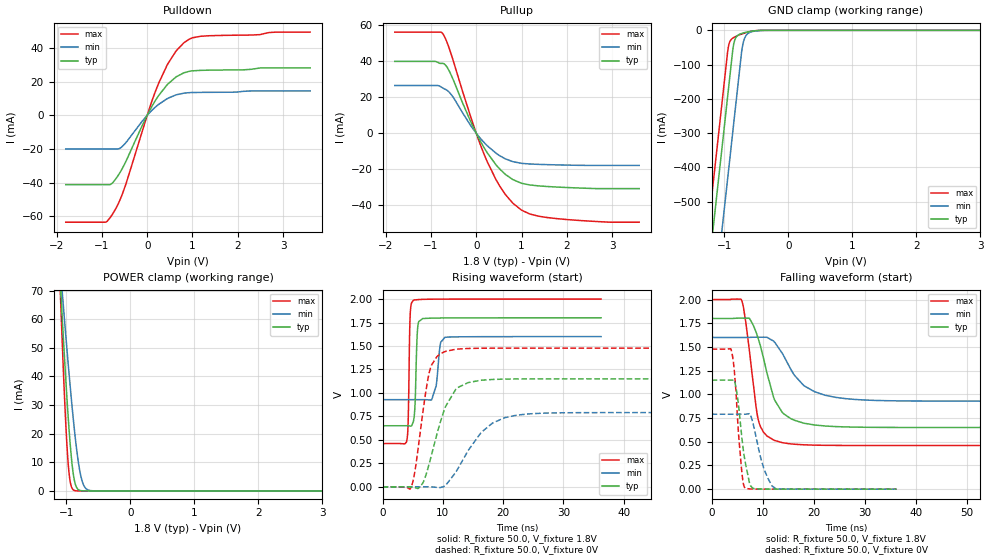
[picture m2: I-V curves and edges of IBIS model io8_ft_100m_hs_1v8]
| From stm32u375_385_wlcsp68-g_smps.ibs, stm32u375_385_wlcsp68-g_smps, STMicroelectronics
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[Model]   io8_ft_100m_hs_1v8
Model_type I/O
Polarity   Non-Inverting
Enable   Active-Low
| CAP_THRESHOLD on pad IOFT is "UDTCAPC" :
| Rising=30.0% of vddiom   Falling=70.0% of vddiom
| C_comp min and max val. don't necessarily correlate with the min and max pvt
| but are the smallest and greatest pad capacitance found.
| var   typ   min   max
C_comp   3.41155pF  3.41004pF  3.47580pF
|C_comp_pullup   1.91894pF  1.83594pF  2.09561pF
|C_comp_pulldown   1.49260pF  1.57410pF  1.38018pF
Vinl = 800.0mV
Vinh = 1.0V
Vmeas = 900.0mV   | Reference voltage for timing measurements
Cref  = 50.0pF   | Timing specification test load capacitance value
Rref  = 1.0MOhm   | Timing specification test load resistance value
Vref  = 990.0mV   | Timing specification test load voltage
[Model Spec]
| TIME_THRESHOLD on pin ZIV11 is "CMOS" :
| Rising=50.0% of vdd   Falling=50.0% of vdd
Vinl 694.50000mV 619.50000mV 778.50000mV
Vinh 1.08350V 957.50000mV 1.18750V
| variable   typ   min   max
[Temperature Range] 25.0 130.0 -40.0
| variable   typ   min   max
[Voltage Range] 1.8V 1.6V 2.0V
| variable   typ   min   max
[POWER Clamp Reference] 1.8V 1.6V 2.0V
| variable   typ   min   max
[GND Clamp Reference] 0V 0V 0V
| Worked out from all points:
|   slope of the pulldown table from 0 to 0.27 V, typ, clamps not added: 21.9 ohm
|   slope of the pullup table from 0 to 0.27 V, typ, clamps not added: 22.8 ohm
|   GND clamp passes 1 mA (typ) near -0.50 V on its own axis
|   POWER clamp passes 1 mA (typ) near -0.83 V on its own axis
|   rising waveform, R_fixture 50.0, V_fixture 1.8V: 20-80 % time 319ps typ, 641ps min, 235ps max; typ from 0.65 V to 1.8 V
|   falling waveform, R_fixture 50.0, V_fixture 1.8V: 20-80 % time 3.79ns typ, 5.6ns min, 2.14ns max; typ from 1.8 V to 0.65 V
|   rising waveform, R_fixture 50.0, V_fixture 0V: 20-80 % time 3.38ns typ, 5.18ns min, 1.96ns max; typ from 0 V to 1.15 V
|   falling waveform, R_fixture 50.0, V_fixture 0V: 20-80 % time 1.6ns typ, 2.3ns min, 1.18ns max; typ from 1.15 V to 0 V
[POWER Clamp]
-1.8V     399.1mA    292.1mA    557.7mA
-1.09V    71.2mA     76.8mA     67.14mA
-1.08V    67.05mA    73.98mA    61.2mA
-1.06V    58.89mA    68.38mA    49.67mA
-1.02V    43.22mA    57.4mA     28.67mA
-980mV    28.81mA    46.77mA    12.28mA
-940mV    16.45mA    36.61mA    3.257mA
-880mV    4.35mA     22.67mA    225.4uA
-820mV    610.4uA    11.29mA    13uA
-770mV    97.5uA     4.87mA     1.193uA
-640mV    753.9nA    196uA      2.499nA
3.6V      0A         0A         0A
[GND Clamp]
-1.8V     -1.64A     -1.88A     -1.509A
-1.24V    -688.2mA   -927.9mA   -557mA
-1.05V    -365.2mA   -604.9mA   -234mA
-950mV    -195.2mA   -434.9mA   -64mA
-930mV    -161.2mA   -400.9mA   -41.59mA
-870mV    -59.19mA   -298.9mA   -22.94mA
-850mV    -36.73mA   -264.9mA   -20.65mA
-770mV    -12.21mA   -128.9mA   -13.73mA
-730mV    -9.139mA   -62.1mA    -10.81mA
-690mV    -6.97mA    -26.33mA   -8.198mA
-530mV    -1.564mA   -2.413mA   -1.407mA
3.6V      1.23nA     159nA      530.1pA
| variable   typ   min   max
[Pullup Reference] 1.8V 1.6V 2.0V
| variable   typ   min   max
[Pulldown Reference] 0V 0V 0V
[Pullup]
-1.8V     39.99mA    26.55mA    56.28mA
-850mV    39.46mA    26.55mA    56.28mA
-740mV    38.87mA    25.21mA    55.4mA
-590mV    34.3mA     22.64mA    46.71mA
-120mV    6.328mA    4.158mA    8.961mA
250mV     -11.14mA   -7.108mA   -16.23mA
440mV     -17.67mA   -11.15mA   -25.97mA
630mV     -22.57mA   -14.06mA   -33.59mA
1V        -27.82mA   -16.74mA   -42.77mA
1.37V     -29.26mA   -17.3mA    -46.1mA
1.74V     -29.87mA   -17.57mA   -47.39mA
3.6V      -30.8mA    -17.88mA   -49.48mA
[Pulldown]
-1.8V     -41.16mA   -19.96mA   -63.43mA
-920mV    -41.16mA   -19.96mA   -63.43mA
-780mV    -40.43mA   -19.96mA   -59.18mA
-620mV    -34.74mA   -19.77mA   -51.3mA
-510mV    -29.46mA   -17.38mA   -43.8mA
0V        0A         0A         0A
250mV     11.64mA    6.428mA    18.87mA
460mV     18.67mA    10.12mA    30.76mA
630mV     22.61mA    12.05mA    37.86mA
810mV     25.21mA    13.14mA    43.03mA
1.18V     26.67mA    13.59mA    46.9mA
3.6V      28.11mA    14.46mA    49.37mA
[Ramp]
dV/dt_r 690.02322mV/3.20375ns 474.36171mV/5.07854ns 886.36558mV/1.95867ns
dV/dt_f 689.75469mV/3.62986ns 403.00334mV/5.43638ns 923.68055mV/2.12778ns
R_load = 50.0
| Removed startup time: 0s 0s 0s  .
| Removed end time: 36.25ns.
[Rising Waveform]
R_fixture   = 50.0
V_fixture   = 1.8V
V_fixture_min = 1.6V
V_fixture_max = 2.0V
0s        650.4mV    928.3mV    460.5mV
4ns       650.4mV    928.3mV    485.9mV
4.25ns    650.2mV    928.3mV    693.7mV
4.6ns     647.3mV    928.3mV    1.852V
5.1ns     690.1mV    928.3mV    1.986V
5.8ns     1.674V     928.3mV    1.994V
6.65ns    1.792V     928.4mV    1.997V
8.15ns    1.797V     926.8mV    1.999V
10.35ns   1.799V     1.593V     2V
36.25ns   1.8V       1.6V       2V
| Removed startup time: 0s 0s 0s  .
| Removed end time: 99.25ns.
[Falling Waveform]
R_fixture   = 50.0
V_fixture   = 1.8V
V_fixture_min = 1.6V
V_fixture_max = 2.0V
0s        1.8V       1.6V       2V
5.85ns    1.804V     1.6V       1.996V
7.45ns    1.799V     1.6V       1.444V
9.15ns    1.587V     1.603V     733.9mV
10.15ns   1.39V      1.602V     603.3mV
12.4ns    936.2mV    1.547V     513.1mV
14.2ns    792.2mV    1.4V       487.5mV
18ns      697.2mV    1.097V     468.1mV
24.3ns    660mV      968.2mV    461.5mV
99.25ns   650.4mV    928.3mV    460.5mV
| Removed startup time: 0s 0s 0s  .
| Removed end time: 99.2ns.
[Rising Waveform]
R_fixture   = 50.0
V_fixture   = 0V
V_fixture_min = 0V
V_fixture_max = 0V
0s        4.649nV    97.48nV    3.434nV
4.65ns    -823.2uV   2.765uV    -14.97mV
5.4ns     -8.809mV   1.906uV    178.2mV
6.6ns     31.54mV    3.369uV    751.9mV
7.8ns     260.6mV    -440.6uV   1.232V
10.45ns   855.4mV    13.84mV    1.443V
12.5ns    1.058V     194mV      1.468V
16.55ns   1.136V     589.6mV    1.476V
22.3ns    1.149V     763.7mV    1.477V
99.2ns    1.15V      790.6mV    1.477V
| Removed startup time: 0s 0s 0s  .
| Removed end time: 36.25ns.
[Falling Waveform]
R_fixture   = 50.0
V_fixture   = 0V
V_fixture_min = 0V
V_fixture_max = 0V
0s        1.15V      790.6mV    1.477V
3.9ns     1.15V      790.6mV    1.457V
4.35ns    1.155V     790.6mV    1.306V
4.85ns    1.05V      790.6mV    970.6mV
5.85ns    589.6mV    790.6mV    226.5mV
6.6ns     285.8mV    790.6mV    10.54mV
8.15ns    7.267mV    691.3mV    1.364mV
10.35ns   1.261mV    200.6mV    597.1uV
12.6ns    648.3uV    6.16mV     297.5uV
36.25ns   1.634uV    11.96uV    82.2nV
